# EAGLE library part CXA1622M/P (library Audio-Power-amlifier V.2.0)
SONY Stereo Power Amplifier/Monaural BTL Power Amplifier
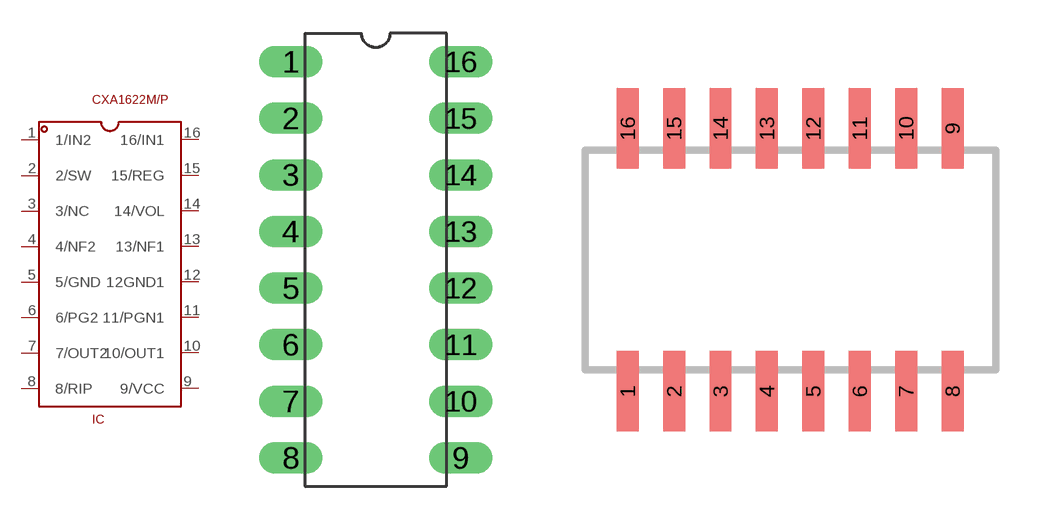
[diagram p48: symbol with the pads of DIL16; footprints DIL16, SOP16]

Designator prefix IC

## CXA1622M/P (DIP16: IC)  [DIL16]
1  1/IN2  in
2  2/SW
3  3/NC  nc
4  4/NF2
5  5/GND  pwr
6  6/PG2  pwr
7  7/OUT2  out
8  8/RIP
9  9/VCC  pwr
10  10/OUT1  out
11  11/PGN1  pwr
12  12GND1  pwr
13  13/NF1
14  14/VOL
15  15/REG
16  16/IN1  in

## CXA1622M/PSOP16  [SOP16]
Pads as for DIL16

## Footprint DIL16 (pad centres in mm)
drill 0.8 pad 1.422 long: 1 -3.81,8.89; 2 -3.81,6.35; 3 -3.81,3.81; 4 -3.81,1.27; 5 -3.81,-1.27; 6 -3.81,-3.81; 7 -3.81,-6.35; 8 -3.81,-8.89; 9 3.81,-8.89; 10 3.81,-6.35; 11 3.81,-3.81; 12 3.81,-1.27; 13 3.81,1.27; 14 3.81,3.81; 15 3.81,6.35; 16 3.81,8.89

## Footprint SOP16 (pad centres in mm)
smd 0.6 x 2.2: 1 -4.445,-3.6; 2 -3.175,-3.6; 3 -1.905,-3.6; 4 -0.635,-3.6; 5 0.635,-3.6; 6 1.905,-3.6; 7 3.175,-3.6; 8 4.445,-3.6; 9 4.445,3.6; 10 3.175,3.6; 11 1.905,3.6; 12 0.635,3.6; 13 -0.635,3.6; 14 -1.905,3.6; 15 -3.175,3.6; 16 -4.445,3.6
